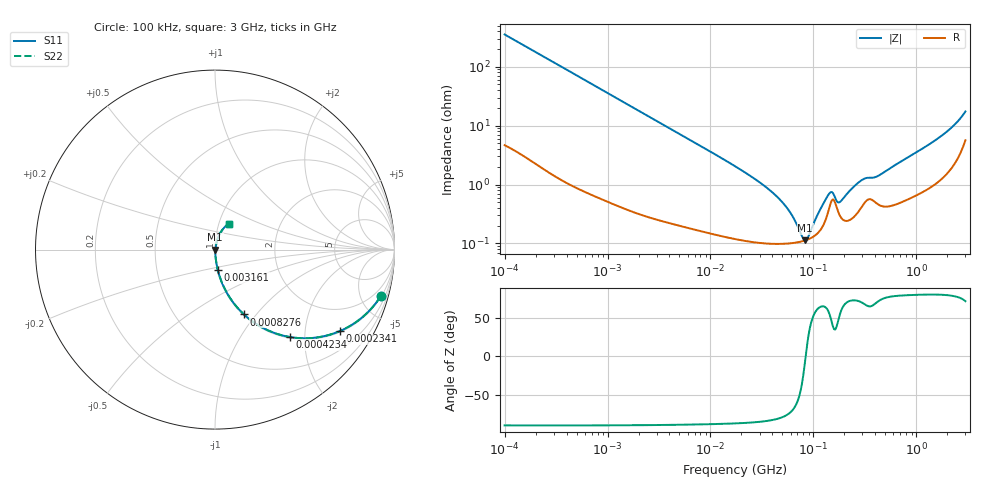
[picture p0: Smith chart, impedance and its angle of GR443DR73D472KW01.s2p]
!Murata Part Number: GR443DR73D472KW01
!These Parameters are Measured in Series Mode Connection
!Data Generated on Mar 13, 2026
!  o--ll--o
!Port1  Port2
!  o------o
!Operation Temp=25[degC], DC Bias Voltage=0[V]
!Freq. Start=100[kHz] Stop=3[GHz] 401[Steps]
# Hz S RI R 50
!Freq.(Hz) S11(Real) S11(Imag) S21(Real) S21(Imag) S12(Real) S12(Imag) S22(Real) S22(Imag)
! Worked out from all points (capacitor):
!   401 points, 100 kHz to 3 GHz, reference 50 ohm
!   read as one part in series: C = 4.5 nF near 105.3 kHz
!   lowest |Z| = 113 mohm at 83.43 MHz (marker M1)
!   series resonance near 84.19 MHz, so ESL is about 790 pH
!   S11 on the Smith chart (normalised r, x): 100 kHz: 1.09, -7.06; 234.1 kHz: 1.04, -3.04; 423.4 kHz: 1.02, -1.69; 827.6 kHz: 1.01, -0.87; 3.161 MHz: 1.00, -0.23; 3 GHz: 1.11, +0.33
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100000  0.9228 -0.2604  0.0772 0.2604  0.0772 0.2604  0.9228 -0.2604
234079  0.6959 -0.4539  0.3041 0.4539  0.3041 0.4539  0.6959 -0.4539
423445  0.4168 -0.4871  0.5832 0.4871  0.5832 0.4871  0.4168 -0.4871
562235  0.2906 -0.4479  0.7094 0.4479  0.7094 0.4479  0.2906 -0.4479
827580  0.1615 -0.3613  0.8385 0.3613  0.8385 0.3613  0.1615 -0.3613
1458987  0.0606 -0.2309  0.9394 0.2309  0.9394 0.2309  0.0606 -0.2309
3161081  0.0153 -0.1124  0.9847 0.1124  0.9847 0.1124  0.0153 -0.1124
1.77727e7  0.00157 -0.0199  0.9984 0.0199  0.9984 0.0199  0.00157 -0.0199
4.732384e7  0.00101 -0.00546  0.999 0.00546  0.999 0.00546  0.00101 -0.00546
5.967813e7  0.00102 -0.00318  0.999 0.00318  0.999 0.00318  0.00102 -0.00318
7.722238e7  0.00109 -0.000802  0.9989 0.000802  0.9989 0.000802  0.00109 -0.000802
8.342988e7  0.00113 -8.49e-05  0.9989 8.49e-05  0.9989 8.49e-05  0.00113 -8.49e-05
8.784301e7  0.00116 0.000401  0.9988 -0.000401  0.9988 -0.000401  0.00116 0.000401
9.738194e7  0.00127 0.00141  0.9987 -0.00141  0.9987 -0.00141  0.00127 0.00141
1.43341e8  0.00414 0.00575  0.9959 -0.00575  0.9959 -0.00575  0.00414 0.00575
1.509232e8  0.00537 0.00514  0.9946 -0.00514  0.9946 -0.00514  0.00537 0.00514
1.807614e8  0.00299 0.00405  0.997 -0.00405  0.997 -0.00405  0.00299 0.00405
2.94964e8  0.00427 0.011  0.9957 -0.011  0.9957 -0.011  0.00427 0.011
4.123589e8  0.00493 0.0127  0.9951 -0.0127  0.9951 -0.0127  0.00493 0.0127
5.475153e8  0.00458 0.0179  0.9954 -0.0179  0.9954 -0.0179  0.00458 0.0179
1.701687e9  0.0155 0.0617  0.9845 -0.0617  0.9845 -0.0617  0.0155 0.0617
3e9  0.0759 0.1442  0.9241 -0.1442  0.9241 -0.1442  0.0759 0.1442
